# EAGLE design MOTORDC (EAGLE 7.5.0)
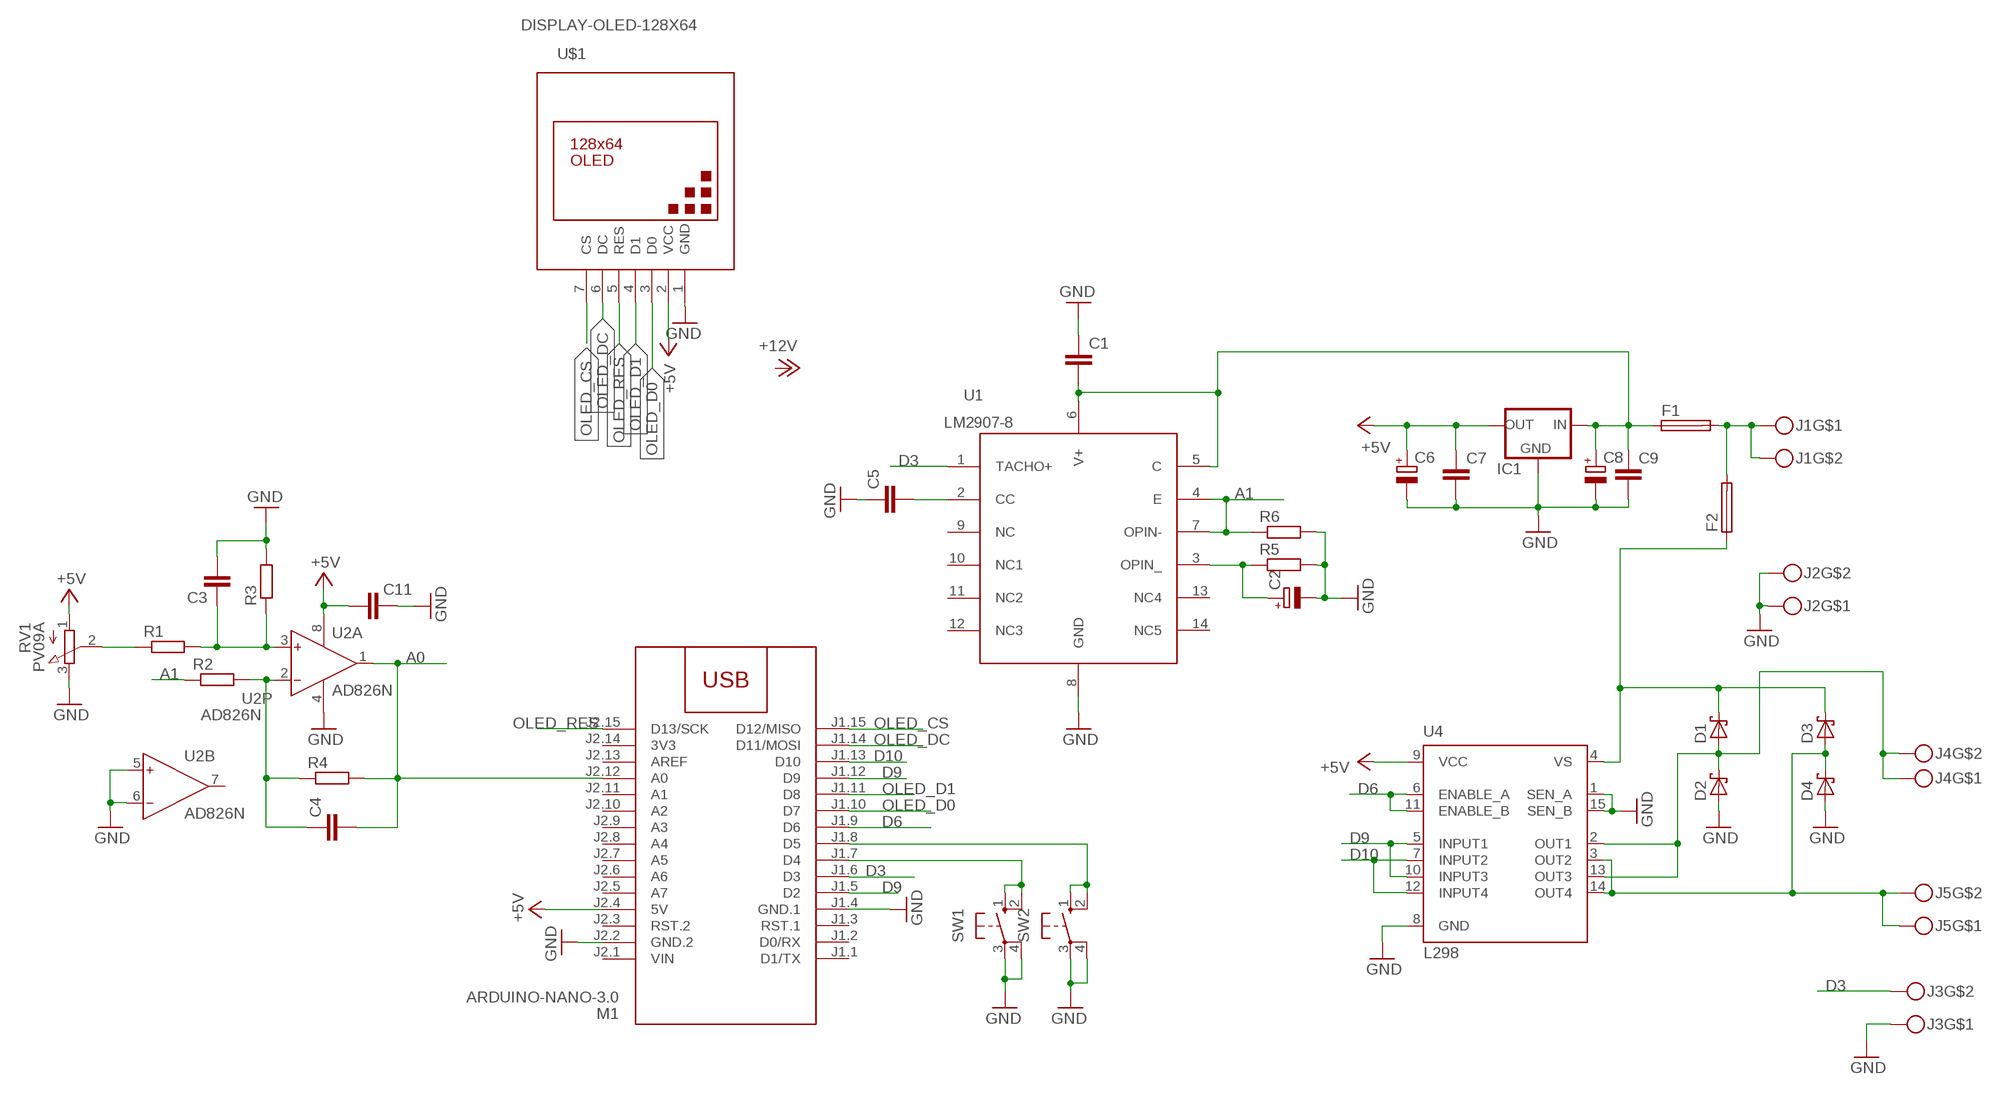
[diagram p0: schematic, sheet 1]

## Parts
C1  C-EUC1206  [C1206]
C2  CPOL-EUE2.5-7  [E2,5-7]
C3  C-EUC1206  [C1206]
C4  C-EUC1206  [C1206]
C5  C-EUC1206  [C1206]
C6  CPOL-EUE2.5-7  [E2,5-7]
C7  C-EUC1206  [C1206]
C8  CPOL-EUE2.5-7  [E2,5-7]
C9  C-EUC1206  [C1206]
C11  C-EUC1206  [C1206]
D1  1N5819-T  [DO41-7.6]
D2  1N5819-T  [DO41-7.6]
D3  1N5819-T  [DO41-7.6]
D4  1N5819-T  [DO41-7.6]
F1  SH22,5  [SH22,5]
F2  SH22,5  [SH22,5]
IC1  78XXL  [78XXL]
J1  MKDSN1,5-2-5,08  [MKDSN1,5-2-5,08]
J2  MKDSN1,5-2-5,08  [MKDSN1,5-2-5,08]
J3  MKDSN1,5-2-5,08  [MKDSN1,5-2-5,08]
J4  MKDSN1,5-2-5,08  [MKDSN1,5-2-5,08]
J5  MKDSN1,5-2-5,08  [MKDSN1,5-2-5,08]
M1  ARDUINO-NANO-3.0  [ARDUINO-NANO-3.0]
R1  R-EU_R1206  [R1206]
R2  R-EU_R1206  [R1206]
R3  R-EU_R1206  [R1206]
R4  R-EU_R1206  [R1206]
R5  R-EU_R1206  [R1206]
R6  R-EU_R1206  [R1206]
RV1  PV09A  [PTV09]
SW1  10-XX  [B3F-10XX]
SW2  10-XX  [B3F-10XX]
U1  LM2907-8  [DIL14]
U2  AD826N  [DIL08]
U4  L298  [MULTIWATT-15]
U$1  DISPLAY-OLED-128X64  [DISPLAY-OLED-128X64]

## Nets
+5V: C6.+ C7.1 C11.2 IC1.OUT M1.J2.4(5V) RV1.1(A) U2.8(P:V+) U4.9(VCC) U$1.2(VCC)
A0: C4.2 M1.J2.12(A0) R4.2 U2.1(A:OUT)
A1: R2.1 R6.1 U1.4(E) U1.7(OPIN-)
D3: J3.2 M1.J1.6(D3) U1.1(TACHO+)
D6: M1.J1.9(D6) U4.6(ENABLE_A) U4.11(ENABLE_B)
D9: M1.J1.5(D2) M1.J1.12(D9) U4.5(INPUT1) U4.10(INPUT3)
D10: M1.J1.13(D10) U4.7(INPUT2) U4.12(INPUT4)
GND: C1.1 C2.- C3.2 C5.1 C6.- C7.2 C8.- C9.2 C11.1 D2.A D4.A IC1.GND J2.1 J2.2 J3.1 M1.J1.4(GND.1) M1.J2.2(GND.2) R3.2 R5.2 R6.2 RV1.3(E) SW1.3(P) SW1.4(P1) SW2.3(P) SW2.4(P1) U1.8(GND) U2.4(P:V-) U2.5(B:IN+) U2.6(B:IN-) U4.1(SEN_A) U4.8(GND) U4.15(SEN_B) U$1.1(GND)
N$1: C1.2 C8.+ C9.1 F1.1 IC1.IN U1.5(C) U1.6(V+)
N$2: C2.+ R5.1 U1.3(OPIN_)
N$3: C4.1 R2.2 R4.1 U2.2(A:IN-)
N$4: F1.2 F2.2 J1.1 J1.2
N$5: D1.A D2.C J4.1 J4.2 U4.2(OUT1) U4.13(OUT3)
N$6: D1.C D3.C F2.1 U4.4(VS)
N$7: C3.1 R1.2 R3.1 U2.3(A:IN+)
N$8: D3.A D4.C J5.1 J5.2 U4.3(OUT2) U4.14(OUT4)
N$9: C5.2 U1.2(CC)
N$10: R1.1 RV1.2(S)
N$11: M1.J1.7(D4) SW1.1(S) SW1.2(S1)
N$13: M1.J1.8(D5) SW2.1(S) SW2.2(S1)
OLED_CS: M1.J1.15(D12/MISO) U$1.7(CS)
OLED_D0: M1.J1.10(D7) U$1.3(D0)
OLED_D1: M1.J1.11(D8) U$1.4(D1)
OLED_DC: M1.J1.14(D11/MOSI) U$1.6(DC)
OLED_RES: M1.J2.15(D13/SCK) U$1.5(RES)
Unconnected: M1.J1.1(D1/TX) M1.J1.2(D0/RX) M1.J1.3(RST.1) M1.J2.3(RST.2) M1.J2.5(A7) M1.J2.6(A6) M1.J2.7(A5) M1.J2.8(A4) M1.J2.9(A3) M1.J2.10(A2) M1.J2.11(A1) M1.J2.13(AREF) U1.9(NC) U1.10(NC1) U1.11(NC2) U1.12(NC3) U1.13(NC4) U1.14(NC5) U2.7(B:OUT)

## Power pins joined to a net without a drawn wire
3V3: M1.J2.14(3V3)
VIN: M1.J2.1(VIN)

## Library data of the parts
C1 C3-C5 C7 C9 C11 = rcl:C-EU: CAPACITOR, European symbol
C2 C6 C8 = rcl:CPOL-EU: POLARIZED CAPACITOR, European symbol
D1-D4 = diode:1N581*: 1.0A SCHOTTKY BARRIER RECTIFIER
F1 F2 = fuse:SH22,5: FUSE HOLDER; MF: SCHURTER; MPN: 0031.8201; OC_FARNELL: 1162740; OC_NEWARK: 96F8317
IC1 = v-reg:78XXL: VOLTAGE REGULATOR
J1-J5 = con-phoenix-508:MKDSN1,5-2-5,08
M1 = diy-modules:ARDUINO-NANO-3.0: Arduino Nano 3.0 and compatible devices More details available here: https://www.arduino.cc/en/Main/ArduinoBoardNano Click here to find device on ebay.com
R1-R6 = rcl:R-EU_: RESISTOR, European symbol
RV1 = pot:PV09A
SW1 SW2 = switch-omron:10-XX: OMRON SWITCH; MPN: B3F-1000; OC_FARNELL: 176432; OC_NEWARK: 36M3542
U1 = analog-devices:LM2907-8: FREQUENCY-VOLTAGE CONVERTER
U2 = analog-devices:AD826: High-Speed, Low-Power Dual Operational Amplifier Source: http://www.analog.com/static/imported-files/data_sheets/AD826.pdf; MF: ALTERA CORPORATION; MPN: AD826ANZ; OC_FARNELL: 1438583; OC_NEWARK: 59K6530
U4 = st-microelectronics:L298: DUAL FULL-BRIDGE DRIVER; MPN: L298N; OC_FARNELL: 1589425; OC_NEWARK: 32M1527
U$1 = diy-modules:DISPLAY-OLED-128X64: 128x64 Dot Matrix OLED Module based on SSD1306 chip Variant with SPI interface More details available here: http://www.instructables.com/id/How-to-use-OLED-display-arduino-module/ SSD1306 datasheet: https://cdn-shop.adafruit.com/datasheets/SSD1306.pdf Click here to find device on ebay.com Note: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

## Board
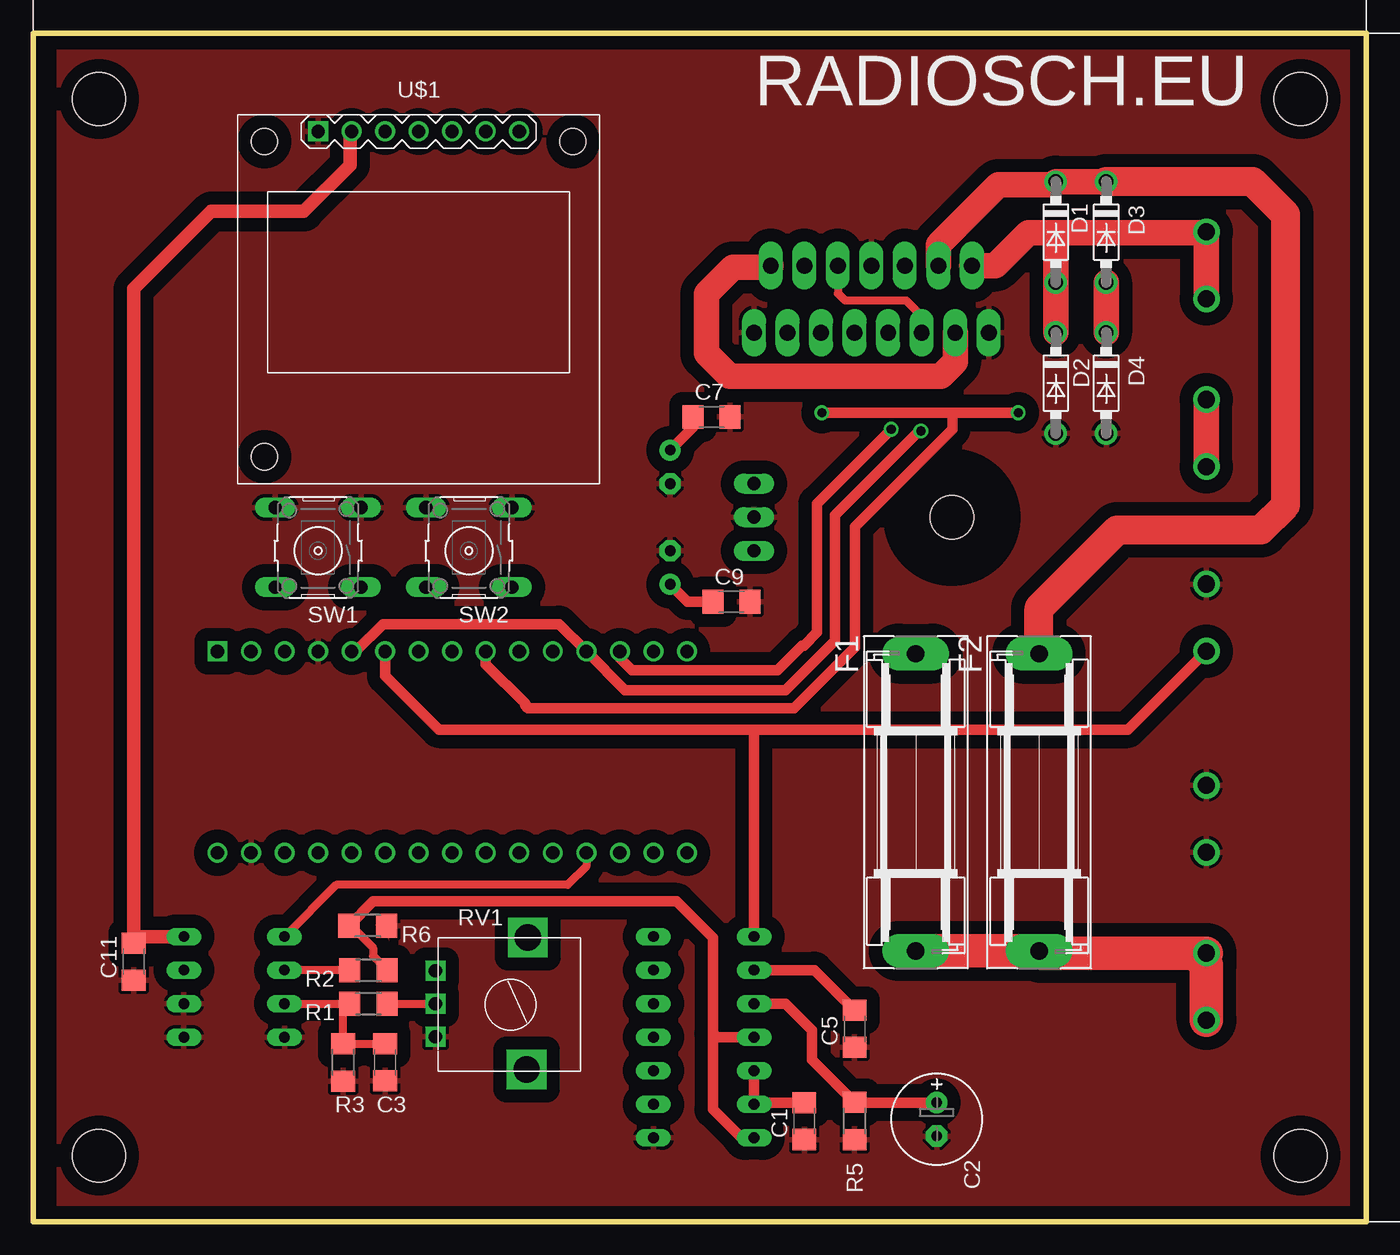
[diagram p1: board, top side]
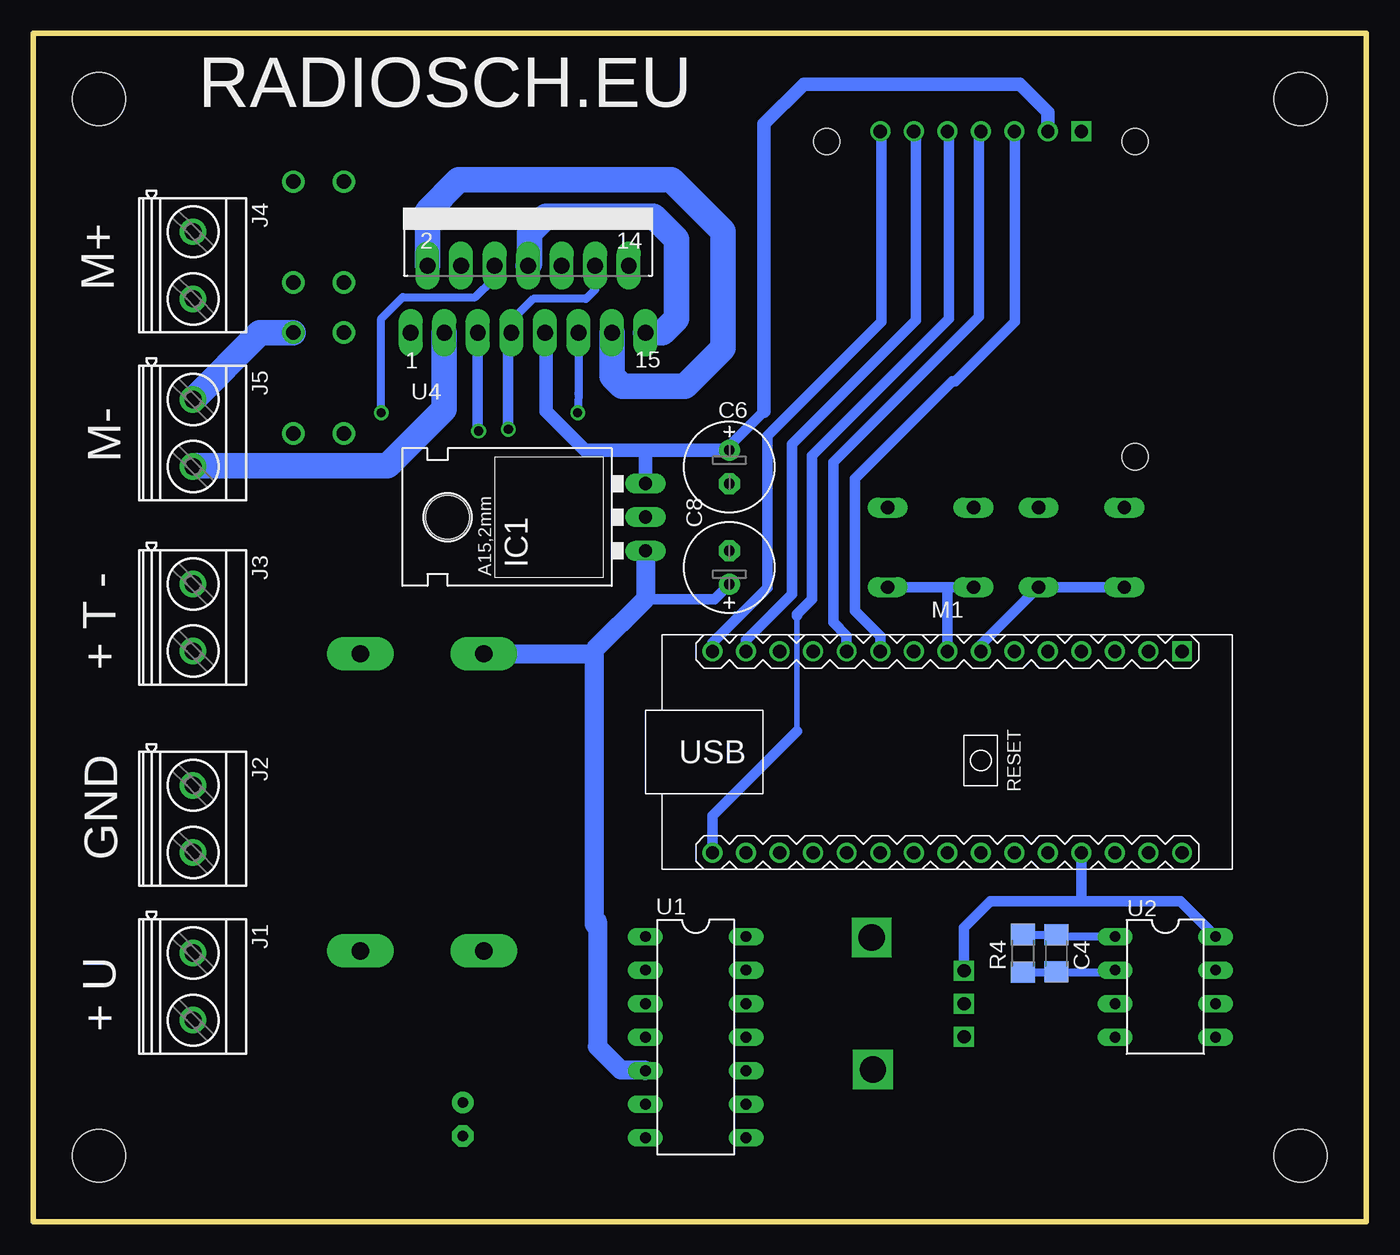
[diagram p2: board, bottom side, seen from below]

Size 101 x 90 mm. Coordinates in mm from the lower left corner, seen from the top.
Outline: 0,0 101,0 101,90 0,90 0,0
Copper layers (1*16): Top 0.035mm / dielectric 1.5mm / Bottom 0.035mm
Design rules "default": minimum track width 10mil, minimum drill 24mil, track to track 8mil, track to pad 8mil, pad to pad 8mil, via to via 8mil, smd to smd 8mil, copper to edge 40mil, drill to drill 8mil, minimum pad ring 10mil, minimum via ring 8mil, stop-mask expansion 4mil, vias tented up to drill 0mil, thermal gap 10mil
Holes 4 mm at 5,5 96,5 5,85 96,85

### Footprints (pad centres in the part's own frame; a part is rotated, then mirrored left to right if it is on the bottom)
C1206 = smd 1.6 x 1.8: 1 -1.4,0; 2 1.4,0
E2,5-7 = drill 0.813 pad 1.6: + -1.27,0 | drill 0.813 pad 1.6 octagon: - 1.27,0
DO41-7.6 = drill 1.1 pad 1.7: A 3.81,0; C -3.81,0
SH22,5 = drill 1.321 pad 2.54 long: 1 -11.252,0; 2 11.252,0
78XXL = drill 1.016 long: GND 0,-3.81; IN -2.54,-3.81; OUT 2.54,-3.81 | hole 3.302: 0,11.176
MKDSN1,5-2-5,08 = drill 1.3 pad 2: 1 -2.561,0.025; 2 2.519,0.025
ARDUINO-NANO-3.0 = drill 1 square: J1.1 17.78,7.62 | drill 1: J1.2 15.24,7.62; J1.3 12.7,7.62; J1.4 10.16,7.62; J1.5 7.62,7.62; J1.6 5.08,7.62; J1.7 2.54,7.62; J1.8 0,7.62; J1.9 -2.54,7.62; J1.10 -5.08,7.62; J1.11 -7.62,7.62; J1.12 -10.16,7.62; J1.13 -12.7,7.62; J1.14 -15.24,7.62; J1.15 -17.78,7.62; J2.1 17.78,-7.62; J2.2 15.24,-7.62; J2.3 12.7,-7.62; J2.4 10.16,-7.62; J2.5 7.62,-7.62; J2.6 5.08,-7.62; J2.7 2.54,-7.62; J2.8 0,-7.62; J2.9 -2.54,-7.62; J2.10 -5.08,-7.62; J2.11 -7.62,-7.62; J2.12 -10.16,-7.62; J2.13 -12.7,-7.62; J2.14 -15.24,-7.62; J2.15 -17.78,-7.62
R1206 = smd 1.6 x 1.803: 1 -1.422,0; 2 1.422,0
PTV09 = drill 1 square: 1 -2.5,0; 2 0,0; 3 2.5,0 | drill 2 square: P$4 -5,7; P$5 5,6.9
B3F-10XX = drill 1.016 long: 1 -3.251,2.761; 2 3.251,2.761; 3 -3.251,-3.261; 4 3.251,-3.261
DIL14 = drill 0.813 long: 1 -7.62,-3.81; 2 -5.08,-3.81; 3 -2.54,-3.81; 4 0,-3.81; 5 2.54,-3.81; 6 5.08,-3.81; 7 7.62,-3.81; 8 7.62,3.81; 9 5.08,3.81; 10 2.54,3.81; 11 0,3.81; 12 -2.54,3.81; 13 -5.08,3.81; 14 -7.62,3.81
DIL08 = drill 0.813 long: 1 -3.81,-3.81; 2 -1.27,-3.81; 3 1.27,-3.81; 4 3.81,-3.81; 5 3.81,3.81; 6 1.27,3.81; 7 -1.27,3.81; 8 -3.81,3.81
MULTIWATT-15 = drill 1.2 long: 1 -8.89,-7.62; 2 -7.62,-2.54; 3 -6.35,-7.62; 4 -5.08,-2.54; 5 -3.81,-7.62; 6 -2.54,-2.54; 7 -1.27,-7.62; 8 0,-2.54; 9 1.27,-7.62; 10 2.54,-2.54; 11 3.81,-7.62; 12 5.08,-2.54; 13 6.35,-7.62; 14 7.62,-2.54; 15 8.89,-7.62
DISPLAY-OLED-128X64 = drill 1 square: 1 -7.62,12.7 | drill 1: 2 -5.08,12.7; 3 -2.54,12.7; 4 0,12.7; 5 2.54,12.7; 6 5.08,12.7; 7 7.62,12.7 | hole 2: -11.684,11.938; 11.684,11.938; -11.684,-11.938

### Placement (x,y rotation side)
C1  58.42,7.62 90 top
C2  68.44,7.75 270 top
C3  26.67,12.06 270 top
C4  23.5,20.32 90 bottom
C5  62.23,14.61 90 top
C6  48.26,57.15 270 bottom
C7  51.39,60.94 0 top
C8  48.26,49.53 90 bottom
C9  52.9,46.94 0 top
C11  7.62,19.68 90 top
D1  77.47,74.93 270 top
D2  77.47,63.5 270 top
D3  81.28,74.93 270 top
D4  81.28,63.5 270 top
F1  66.86,31.75 270 top
F2  76.2,31.75 270 top
IC1  58.42,53.34 90 bottom
J1  88.9,17.78 270 bottom
J2  88.9,30.48 270 bottom
J3  88.9,45.72 270 bottom
J4  88.9,72.39 270 bottom
J5  88.9,59.69 270 bottom
M1  31.75,35.56 0 bottom
R1  25.4,16.51 180 top
R2  25.4,19.05 180 top
R3  23.5,12.06 270 top
R4  26.04,20.32 90 bottom
R5  62.23,7.62 270 top
R6  25.35,22.41 0 top
RV1  30.48,16.51 270 top
SW1  21.59,50.8 180 top
SW2  33.02,50.8 180 top
U1  50.8,13.97 270 bottom
U2  15.24,17.78 270 bottom
U4  63.5,74.93 0 bottom
U$1  29.21,69.85 0 top

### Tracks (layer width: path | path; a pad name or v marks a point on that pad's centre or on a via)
+5V
  Top 0.813: C7.1 49.99,60.15 C6.+
  Top 1.016: U$1.2 24,82.42 24,80 20.5,76.5 13.5,76.5 7.62,70.62 C11.2 8.12,21.59 U2.8
  Bottom 0.813: RV1.1 30.48,22.27 28.5,24.25 21.75,24.25 | 21.75,24.25 14.09,24.25 U2.8 | M1.J2.4 21.59,24.41 21.75,24.25 | 48.07,58.61 48.07,58.93 45.62,61.38
  Bottom 1.016: 45.62,61.38 45.62,83.12 42.62,86.12 26.25,86.12 24.12,84 U$1.2 | 48.07,58.61 C6.+ 54.88,58.42 | 54.88,58.42 59.17,58.42 62.12,61.38 62.12,67.2 U4.9 | IC1.OUT 54.61,58.16 54.88,58.42
A0
  Top 0.61: M1.J2.12 41.91,26.91 40.5,25.5 22.96,25.5 U2.1
  Bottom 0.61: R4.2 23.52,21.74 C4.2 23.36,21.59 U2.1
A1
  Top 0.61: R6.1 24.09,22.41 25.75,20.75 25.75,20.12 R2.1
  Top 0.813: R6.1 25.77,24.25 48.75,24.25 51.5,21.5 51.5,14.25 | 51.5,14.25 51.5,8.5 53.5,6.5 54.46,6.5 U1.7 | U1.4 51.78,13.97 51.5,14.25
D3
  Top 0.813: M1.J1.6 26.67,41.33 30.75,37.25 54.38,37.25 | J3.2 82.92,37.25 54.38,37.25 | U1.1 54.61,37.02 54.38,37.25
D6  (via drill 0.7)
  Top 0.813: v59.75,61.25 69.75,61.25 | 69.75,61.25 v74.62,61.25 | M1.J1.9 34.29,42.21 37.25,39.25 37.25,39.12 37.5,38.88 57.62,38.88 62.25,43.5 62.25,52.62 69.62,60 69.62,61.12 69.75,61.25
  Bottom 0.61: U4.11 59.69,62.69 v59.75,61.25 | v74.62,61.25 74.62,68.38 73,70 67.5,70 66.12,71.38 66.12,72.31 U4.6
D9  (via drill 0.7)
  Top 0.61: U4.10 60.96,70.29 61.5,69.75 66.12,69.75 67.31,68.56 U4.5
  Top 0.813: M1.J1.5 24.43,43.18 26.5,45.25 39.84,45.25 M1.J1.12 44.84,40.25 57,40.25 60.75,44 60.75,53.5 67.12,59.88 v67.25,59.88
  Bottom 0.813: U4.5 67.31,59.94 v67.25,59.88
D10  (via drill 0.7)
  Top 0.813: M1.J1.13 44.45,42.67 45.38,41.75 56.38,41.75 58.25,43.62 58.38,43.62 59.38,44.62 59.38,54.38 v65,60
  Bottom 0.61: U4.12 58.42,70.58 59.12,69.88 63.12,69.88 64.75,68.25 64.75,67.33 U4.7
  Bottom 0.813: v65,60 65,67.08 U4.7
GND
  Bottom 0.813: 48.19,55.81 C6.-
  Bottom 1.93: U4.15 53.31,67.31 52.25,68.38 52.25,74.38 54,76.12 62.12,76.12 63.38,74.88 63.38,72.52 U4.8
  pour Top (isolate 1): 2,89 100.5,89.12 100.5,1.12 2,1
N$1
  Top 0.813: C1.2 54.74,9.02 U1.6 U1.5 | C9.1 49.58,46.94 C8.+
  Bottom 0.813: 54.61,47.14 49.38,47.14 C8.+
  Bottom 1.422: 58.25,22.75 58.25,22.25 | 58.25,22.25 58.25,13.25 56.5,11.5 54.68,11.5 U1.5 | IC1.IN 54.61,47.14 58.5,43.25 58.5,43 | 58.5,43 58.5,22.5 58.25,22.25 | F1.1 58.5,43
N$2
  Top 0.813: U1.3 56.99,16.51 59,14.5 59,12.27 R5.1 62.25,9.03 C2.+
N$3
  Top 0.61: R2.2 U2.2
  Bottom 0.61: R4.1 23.52,18.9 | 23.52,18.9 C4.1 | 23.52,18.9 19.2,18.9 U2.2
N$4
  Top 2.54: J1.1 88,20.34 | 88,20.34 76.36,20.34 F2.2 F1.2 | J1.2 88.88,19.47 88,20.34
N$5
  Top 1.93: U4.2 72.89,72.39 75.38,74.88 77.75,74.88 | 77.75,74.88 88.8,74.88 J4.1 J4.2 | 77.75,74.88 77.47,74.59 D1.A D2.C
  Bottom 1.93: U4.13 57.15,64.03 56.38,63.25 51.62,63.25 48.75,66.12 48.75,75 52.62,78.88 68.75,78.88 71.12,76.5 U4.2
N$6
  Top 1.93: U4.4 68.58,73.95 73.12,78.5 77.23,78.5 D1.C D3.C
  Top 2.184: F2.1 76.2,46.45 82.12,52.38 93,52.38 94.88,54.25 94.88,76.25 92.38,78.75 D3.C
N$7
  Top 0.61: U2.3 R1.2 23.5,16.03 R3.1 26.65,13.49 C3.1
N$8
  Top 1.93: D3.A D4.C | J5.2 J5.1 | U4.14 55.74,72.25 53,72.25 51,70.25 51,65.75 52.75,64 68.75,64 69.85,65.1 U4.3
  Bottom 1.93: U4.3 69.85,61.52 74.12,57.25 88.8,57.25 J5.2 | D4.C 83.82,67.31 J5.1
N$9
  Top 0.813: U1.2 59.19,19.05 C5.2
N$10
  Top 0.61: R1.1 RV1.2
N$11
  Bottom 0.813: SW1.2 SW1.1 29.21,43.67 M1.J1.7
N$13
  Bottom 0.813: SW2.2 31.75,48.04 | 31.75,48.04 SW2.1 | M1.J1.8 31.75,48.04
OLED_CS
  Bottom 0.813: M1.J1.15 49.53,43.84 45.38,48 45.38,59.5 36.75,68.12 36.75,82.47 U$1.7
OLED_D0
  Bottom 0.813: M1.J1.10 36.83,44.33 38.75,46.25 38.75,56.25 31.38,63.62 31.12,63.62 26.62,68.12 26.62,82.5 U$1.3
OLED_D1
  Bottom 0.813: M1.J1.11 39.37,44.37 40.38,45.38 40.38,57.5 29.38,68.5 29.38,82.39 U$1.4
OLED_DC
  Bottom 0.813: M1.J1.14 46.99,44.01 43.5,47.5 43.5,58.88 34.12,68.25 34.12,82.39 U$1.6
OLED_RES
  Bottom 0.406: 43.12,37.12 43.12,45.88
  Bottom 0.813: M1.J2.15 49.53,30.72 43.12,37.12 | 43.12,45.88 43.12,46 42,47.12 42,58 31.62,68.38 31.62,82.42 U$1.5

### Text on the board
tPlace: RADIOSCH.EU
bPlace: RADIOSCH.EU | M+ | M- | + T - | GND | + U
